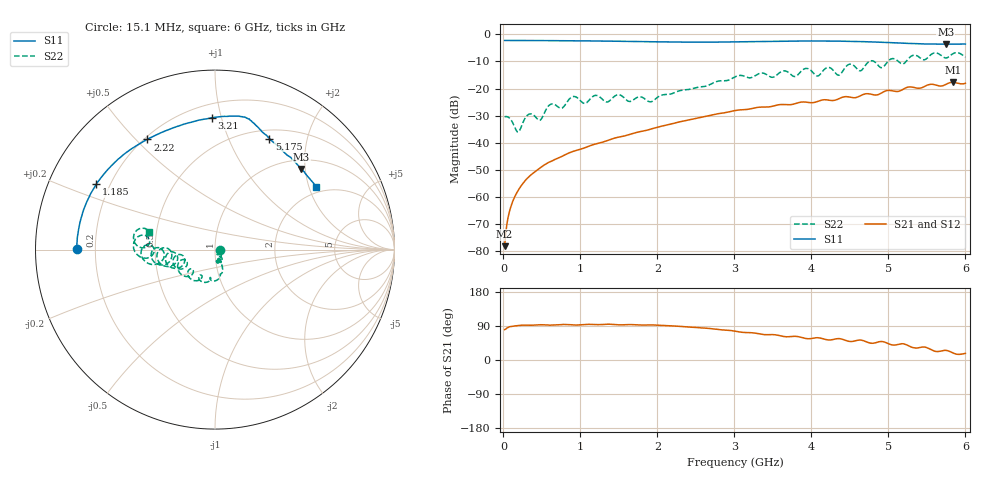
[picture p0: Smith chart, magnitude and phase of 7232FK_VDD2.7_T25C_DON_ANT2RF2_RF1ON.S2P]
!Agilent Technologies,E5071C,MY46417908,A.11.23
!Date: Fri Mar 03 11:31:17 2017
!Data & Calibration Information:
!Freq	S11:SOLT2(ON)	S21:SOLT2(ON)	S12:SOLT2(ON)	S22:SOLT2(ON)
!PortZ  Port1:50+j0  Port2:50+j0
!Above PortZ is port z conversion or system Z0 setting when saving the data.
!When reading, reference impedance value at option line is always used.
# Hz S dB R 50
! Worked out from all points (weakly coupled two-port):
!   400 points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, 15.1 MHz to 6 GHz, reference 50 ohm
!   highest |S21| = -17.70 dB at 5.835 GHz (marker M1); lowest = -78.1 dB at 15.1 MHz (marker M2)
!   lowest |S11| = -3.6 dB at 5.745 GHz (marker M3), VSWR 4.84, Z = 60.3 + j95.3 ohm
!   |S11| at or under -10 dB: nowhere
!   |S22| runs from -36.0 to -6.8 dB; largest |S21 - S12| = 0.0028
!   S11 on the Smith chart (normalised r, x): 15.1 MHz: 0.13, +0.00; 1.185 GHz: 0.15, +0.25; 2.22 GHz: 0.21, +0.54; 3.21 GHz: 0.29, +0.93; 5.175 GHz: 0.61, +1.43; 6 GHz: 1.81, +2.24
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1.509975e7  -2.25 179.6  -78.13 80.1  -77.96 81.7  -30.40 -5.2
9.00985e7  -2.26 177.9  -64.12 88.1  -64.11 88.1  -31.26 -35.2
1.950968e8  -2.27 175.5  -57.38 91.0  -57.39 91.1  -36.03 -29.5
2.700955e8  -2.28 173.9  -54.37 91.9  -54.37 92.2  -31.49 -22.7
4.80092e8  -2.30 168.9  -49.20 93.0  -49.19 93.1  -31.63 -53.1
6.0009e8  -2.32 166.0  -47.07 91.9  -47.07 91.9  -26.04 -45.1
9.00085e8  -2.37 158.6  -43.22 92.7  -43.23 92.8  -22.99 -58.6
1.020083e9  -2.39 155.5  -42.21 93.2  -42.23 93.0  -25.02 -71.8
1.18508e9  -2.44 151.2  -40.53 93.4  -40.52 93.4  -22.58 -65.7
2.010066e9  -2.76 128.1  -34.18 91.8  -34.19 91.8  -23.05 -62.1
2.220063e9  -2.85 121.5  -32.76 89.8  -32.76 89.9  -21.52 -61.5
3.01505e9  -2.77 96.6  -28.08 75.8  -28.06 75.9  -15.59 -83.8
3.210046e9  -2.67 91.5  -27.47 72.1  -27.46 72.1  -16.03 -99.1
4.005033e9  -2.44 78.2  -25.23 56.9  -25.21 56.7  -13.63 -161.7
4.350028e9  -2.51 75.0  -23.83 56.4  -23.87 56.4  -15.08 -164.7
4.485025e9  -2.57 74.1  -23.08 49.3  -23.06 49.0  -11.11 -162.8
4.635023e9  -2.67 72.6  -22.67 52.7  -22.64 52.5  -13.46 -168.5
5.010016e9  -3.04 67.6  -20.66 42.2  -20.60 42.4  -9.50 -166.3
5.175014e9  -3.24 63.9  -20.52 43.0  -20.50 43.2  -10.92 -176.5
5.745004e9  -3.64 43.0  -18.49 25.5  -18.44 26.2  -8.72 173.3
5.835003e9  -3.64 39.4  -17.70 18.9  -17.61 19.9  -7.20 176.9
6e9  -3.57 31.5  -18.04 17.4  -18.00 18.3  -8.41 164.7
